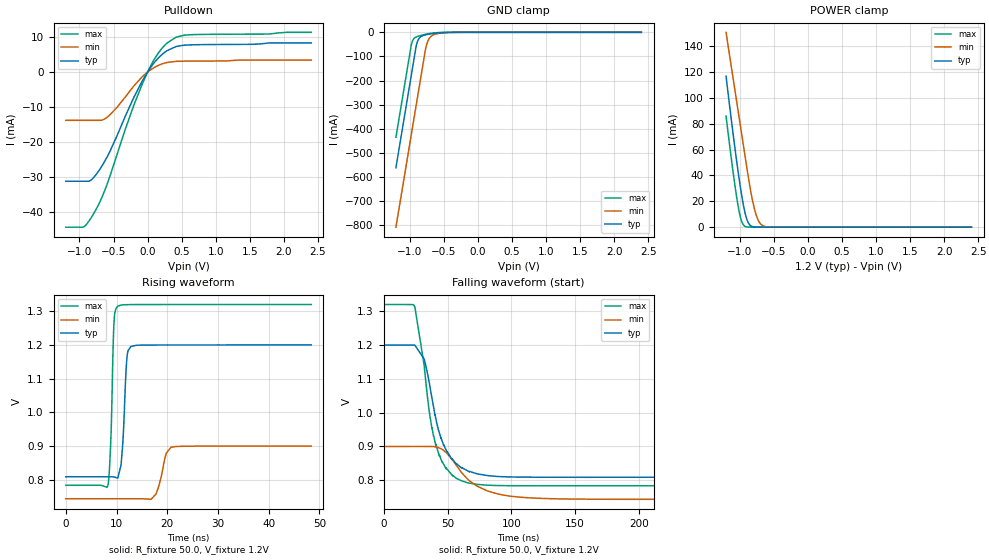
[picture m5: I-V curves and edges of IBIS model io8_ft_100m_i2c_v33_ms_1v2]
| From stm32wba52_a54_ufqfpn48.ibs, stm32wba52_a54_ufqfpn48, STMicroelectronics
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[Model]   io8_ft_100m_i2c_v33_ms_1v2
Model_type I/O_open_drain
Polarity   Non-Inverting
Enable   Active-Low
| CAP_THRESHOLD on pad IOFT is "UDTCAPC" :
| Rising=30.0% of vddiom   Falling=70.0% of vddiom
| C_comp min and max val. don't necessarily correlate with the min and max pvt
| but are the smallest and greatest pad capacitance found.
| var   typ   min   max
C_comp   1.75955pF  1.58205pF  1.89750pF
|C_comp_pulldown   1.75955pF  1.58205pF  1.89750pF
Vinl = 450.0mV
Vinh = 660.0mV
Vmeas = 600.0mV   | Reference voltage for timing measurements
Cref  = 50.0pF   | Timing specification test load capacitance value
Rref  = 1.0MOhm   | Timing specification test load resistance value
Vref  = 660.0mV   | Timing specification test load voltage
[Model Spec]
| TIME_THRESHOLD on pin ZII2CV11 is "CMOS" :
| Rising=50.0% of vdd   Falling=50.0% of vdd
Vinl 436.50000mV 342.50000mV 466.50000mV
Vinh 753.50000mV 549.50000mV 839.50000mV
| variable   typ   min   max
[Temperature Range] 25.0 140.0 -40.0
| variable   typ   min   max
[Voltage Range] 1.2V 900.0mV 1.32V
| variable   typ   min   max
[POWER Clamp Reference] 1.2V 900.0mV 1.32V
| variable   typ   min   max
[GND Clamp Reference] 0V 0V 0V
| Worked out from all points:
|   slope of the pulldown table from 0 to 0.18 V, typ, clamps not added: 40.6 ohm
|   GND clamp passes 1 mA (typ) near -0.51 V on its own axis
|   POWER clamp passes 1 mA (typ) near -0.83 V on its own axis
|   rising waveform, R_fixture 50.0, V_fixture 1.2V: 20-80 % time 745ps typ, 1.43ns min, 565ps max; typ from 0.809 V to 1.2 V
|   falling waveform, R_fixture 50.0, V_fixture 1.2V: 20-80 % time 15.2ns typ, 25.5ns min, 13.4ns max; typ from 1.2 V to 0.809 V
[POWER Clamp]
-1.2V     116.7mA    150.7mA    85.92mA
-1.06V    57.23mA    102.6mA    28.68mA
-1.02V    41.75mA    88.91mA    15.5mA
-980mV    27.6mA     75.18mA    5.935mA
-920mV    10.75mA    54.6mA     597.6uA
-870mV    3.065mA    37.68mA    60.82uA
-820mV    594.6uA    22.85mA    5.912uA
-770mV    99.71uA    11.47mA    572nA
-730mV    23.34uA    5.552mA    88.29nA
-680mV    3.779uA    1.833mA    8.565nA
-510mV    7.889nA    23.13uA    53.67pA
2.4V      0A         0A         0A
[GND Clamp]
-1.2V     -561.6mA   -807.5mA   -434.8mA
-980mV    -187.6mA   -433.5mA   -60.76mA
-960mV    -153.6mA   -399.5mA   -38.21mA
-900mV    -54.17mA   -297.5mA   -18.87mA
-870mV    -29.55mA   -246.5mA   -15.73mA
-830mV    -17.05mA   -178.5mA   -12.57mA
-760mV    -9.921mA   -62.77mA   -8.045mA
-730mV    -8.191mA   -35.56mA   -6.403mA
-680mV    -5.826mA   -15.57mA   -4.089mA
-580mV    -2.43mA    -5.043mA   -1.157mA
-330mV    -11.72uA   -245.5uA   -300.5nA
2.4V      872pA      1.056uA    338.3pA
| variable   typ   min   max
[Pullup Reference] 1.2V 900.0mV 1.32V
| variable   typ   min   max
[Pulldown Reference] 0V 0V 0V
[Pulldown]
-1.2V     -31.2mA    -13.81mA   -44.3mA
-940mV    -31.2mA    -13.81mA   -44.26mA
-850mV    -31.11mA   -13.81mA   -42.26mA
-760mV    -29.39mA   -13.81mA   -39.38mA
-660mV    -26.52mA   -13.68mA   -35.32mA
-550mV    -22.55mA   -12.17mA   -29.6mA
-330mV    -12.74mA   -7.204mA   -16.5mA
-80mV     -2.622mA   -1.37mA    -3.49mA
110mV     2.963mA    1.428mA    3.999mA
290mV     6.144mA    2.737mA    8.347mA
540mV     7.674mA    3.096mA    10.53mA
2.4V      8.312mA    3.389mA    11.33mA
[Ramp]
dV/dt_r 234.64965mV/734.73185ps 93.74419mV/1.39435ns 321.76572mV/560.44232ps
dV/dt_f 234.65981mV/15.08221ns 93.76342mV/24.5418ns 321.77307mV/12.36102ns
R_load = 50.0
| Removed startup time: 0s 0s 0s  .
| Removed end time: 48.4ns.
[Rising Waveform]
R_fixture   = 50.0
V_fixture   = 1.2V
V_fixture_min = 900.0mV
V_fixture_max = 1.32V
0s        808.9mV    743.7mV    783.7mV
8.25ns    808.9mV    743.7mV    780.7mV
8.9ns     809mV      743.7mV    926.1mV
9.5ns     808.4mV    743.7mV    1.265V
10.25ns   804.7mV    743.7mV    1.315V
11.2ns    900.5mV    743.7mV    1.319V
12.05ns   1.16V      743.7mV    1.319V
12.85ns   1.196V     743.7mV    1.32V
20.75ns   1.2V       896.5mV    1.32V
48.4ns    1.2V       900mV      1.32V
| Removed startup time: 0s 0s 0s  .
| Removed end time: 398.4ns.
[Falling Waveform]
R_fixture   = 50.0
V_fixture   = 1.2V
V_fixture_min = 900.0mV
V_fixture_max = 1.32V
0s        1.2V       900mV      1.32V
24.4ns    1.2V       900mV      1.313V
31.65ns   1.159V     900mV      1.142V
36.45ns   1.073V     899.9mV    984.1mV
40.75ns   984.5mV    898.7mV    905.1mV
49.45ns   884.6mV    880.2mV    834.1mV
61.2ns    837.4mV    821.9mV    798.2mV
81.3ns    813.8mV    768.4mV    785.4mV
113.9ns   809.2mV    748.1mV    783.7mV
398.4ns   808.9mV    743.7mV    783.7mV
